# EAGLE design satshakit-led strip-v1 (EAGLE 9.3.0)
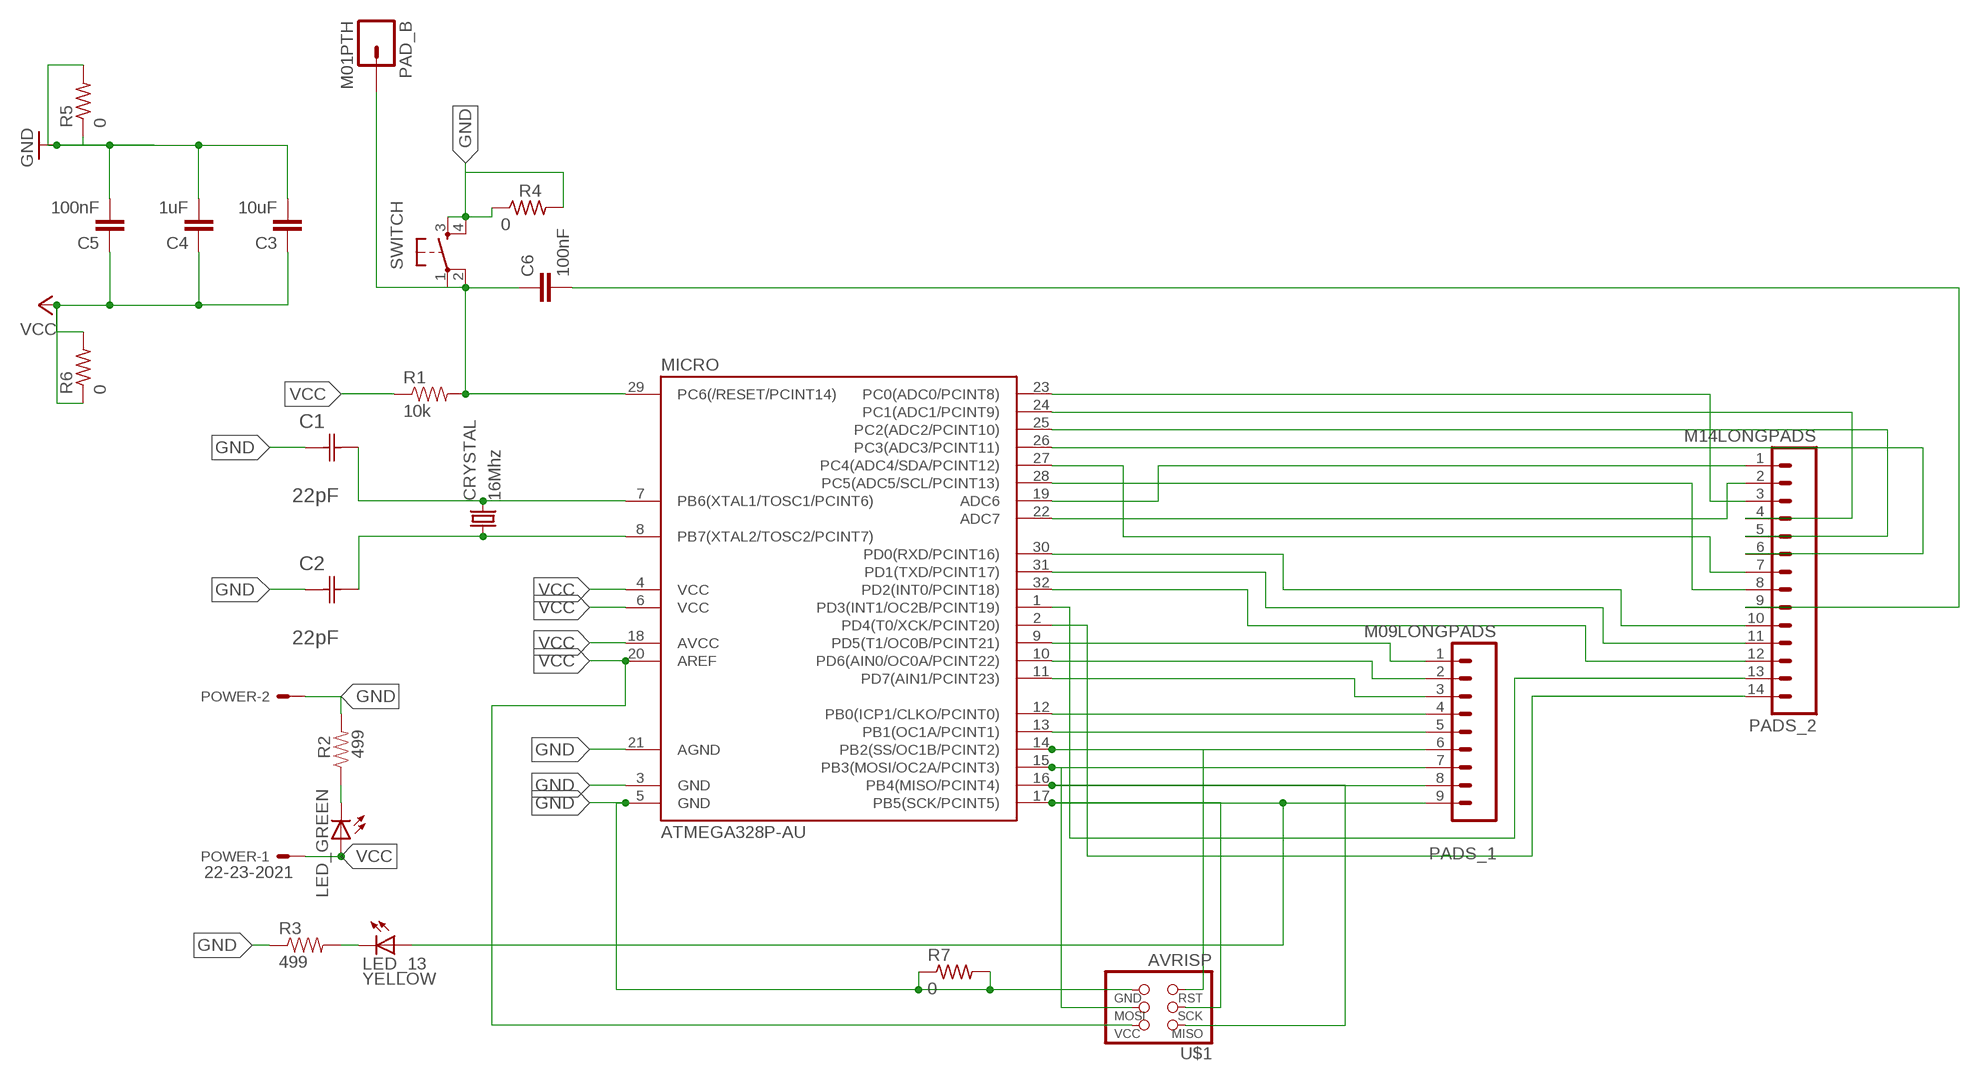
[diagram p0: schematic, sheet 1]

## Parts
C1  22pF  0612ZC225MAT2A  [CAPC3216X178N]
C2  22pF  0612ZC225MAT2A  [CAPC3216X178N]
C3  10uF  CAP1206  [1206]
C4  1uF  CAP1206  [1206]
C5  100nF  CAP1206  [1206]
C6  100nF  CAP1206  [1206]
CRYSTAL  16Mhz  CSM-7X-DU  [CSM-7X-DU]
LED_13  YELLOW  LED1206  [1206]
LED_GREEN  LED1206  [1206]
MICRO  ATMEGA328P-AU  ATMEGA48/88/168-AU  [TQFP32-08]
PAD_B  M01PTH  [1X01]
PADS_1  M09LONGPADS  [1X09_LONGPADS]
PADS_2  M14LONGPADS  [1X14-LONGPADS]
POWER  22-23-2021  [22-23-2021]
R1  10k  RESISTOR1206  [1206]
R2  499  RESISTOR1206  [1206]
R3  499  RESISTOR1206  [1206]
R4  0  RES-US1206  [R1206]
R5  0  RES-US1206FAB  [R1206FAB]
R6  0  RES-US1206FAB  [R1206FAB]
R7  0  RES-US1206FAB  [R1206FAB]
SWITCH  6MM_SWITCH6MM_SWITCH  [6MM_SWITCH]
U$1  AVRISP  [2X03]

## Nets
GND: C1.1(C1) C2.1(C1) C3.2 C4.2 C5.2 MICRO.3(GND) MICRO.5(GND) MICRO.21(AGND) POWER.2 R2.2 R3.1 R4.1 R4.2 R5.1 R5.2 R7.1 R7.2 SWITCH.3(S) SWITCH.4(S1) U$1.6(GND)
N$1: MICRO.9(PD5(T1/OC0B/PCINT21)) PADS_1.1
N$2: C1.2(C2) CRYSTAL.2 MICRO.7(PB6(XTAL1/TOSC1/PCINT6))
N$3: C6.2 PADS_2.9
N$4: MICRO.10(PD6(AIN0/OC0A/PCINT22)) PADS_1.2
N$5: MICRO.11(PD7(AIN1/PCINT23)) PADS_1.3
N$6: MICRO.12(PB0(ICP1/CLKO/PCINT0)) PADS_1.4
N$7: MICRO.13(PB1(OC1A/PCINT1)) PADS_1.5
N$8: MICRO.14(PB2(SS/OC1B/PCINT2)) PADS_1.6 U$1.5(RST)
N$9: C2.2(C2) CRYSTAL.1 MICRO.8(PB7(XTAL2/TOSC2/PCINT7))
N$10: MICRO.15(PB3(MOSI/OC2A/PCINT3)) PADS_1.7 U$1.4(MOSI)
N$11: MICRO.16(PB4(MISO/PCINT4)) PADS_1.8 U$1.1(MISO)
N$12: LED_13.1(A) MICRO.17(PB5(SCK/PCINT5)) PADS_1.9 U$1.3(SCK)
N$13: MICRO.19(ADC6) PADS_2.1
N$14: MICRO.22(ADC7) PADS_2.2
N$15: MICRO.23(PC0(ADC0/PCINT8)) PADS_2.3
N$16: MICRO.24(PC1(ADC1/PCINT9)) PADS_2.4
N$17: MICRO.25(PC2(ADC2/PCINT10)) PADS_2.5
N$18: MICRO.26(PC3(ADC3/PCINT11)) PADS_2.6
N$19: MICRO.27(PC4(ADC4/SDA/PCINT12)) PADS_2.7
N$20: MICRO.30(PD0(RXD/PCINT16)) PADS_2.10
N$21: MICRO.31(PD1(TXD/PCINT17)) PADS_2.11
N$22: MICRO.32(PD2(INT0/PCINT18)) PADS_2.12
N$23: MICRO.1(PD3(INT1/OC2B/PCINT19)) PADS_2.13
N$24: MICRO.2(PD4(T0/XCK/PCINT20)) PADS_2.14
N$25: MICRO.28(PC5(ADC5/SCL/PCINT13)) PADS_2.8
N$26: LED_GREEN.2(C) R2.1
N$27: LED_13.2(C) R3.2
N$28: C6.1 MICRO.29(PC6(/RESET/PCINT14)) PAD_B.1 R1.2 SWITCH.1(P) SWITCH.2(P1)
VCC: C3.1 C4.1 C5.1 LED_GREEN.1(A) MICRO.4(VCC) MICRO.6(VCC) MICRO.18(AVCC) MICRO.20(AREF) POWER.1 R1.1 R6.1 R6.2 U$1.2(VCC)

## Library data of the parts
C1 C2 = AVX_By_element14_Batch_1:0612ZC225MAT2A: Capacitor 1206; MPN: 0612ZC225MAT2A; OC_FARNELL: -; OC_NEWARK: 12N3209; SUPPLIER: AVX; TOLERANCE: ±20%; VALUE: 2.2µF; VOLTAGERATING: 10V
C3-C6 = 01_SparkFun:CAP: Capacitor
CRYSTAL = 01_FAB_Hello:CSM-7X-DU: SMD CRYSTAL; OC_FARNELL: unknown; OC_NEWARK: unknown
LED_13 LED_GREEN = 01_FAB_Hello:LED
MICRO = atmega8:ATMEGA48/88/168
PAD_B = 01_SparkFun:M01: Header 1
PADS_1 = 01_SparkFun:M09: Header 9 Standard 9-pin 0.1" header. Use with straight break away headers (SKU : PRT-00116), right angle break away headers (PRT-00553), swiss pins (PRT-00743), machine pins (PRT-00117), and female headers (PRT-00115).
PADS_2 = 01_SparkFun:M14: Header 14 Standard 14-pin 0.1" header. Use with straight break away headers (SKU : PRT-00116), right angle break away headers (PRT-00553), swiss pins (PRT-00743), machine pins (PRT-00117), and female headers (PRT-00115).
POWER = con-molex:22-23-2021: .100" (2.54mm) Center Header - 2 Pin; MF: MOLEX; MPN: 22-23-2021; OC_FARNELL: 1462926; OC_NEWARK: 25C3832
R1-R3 = 01_SparkFun:RESISTOR: Resistor
R4-R7 = fab:RES-US: Resistor (US Symbol)
SWITCH = 01_FAB_Hello:6MM_SWITCH: OMRON SWITCH
U$1 = fab:AVRISP

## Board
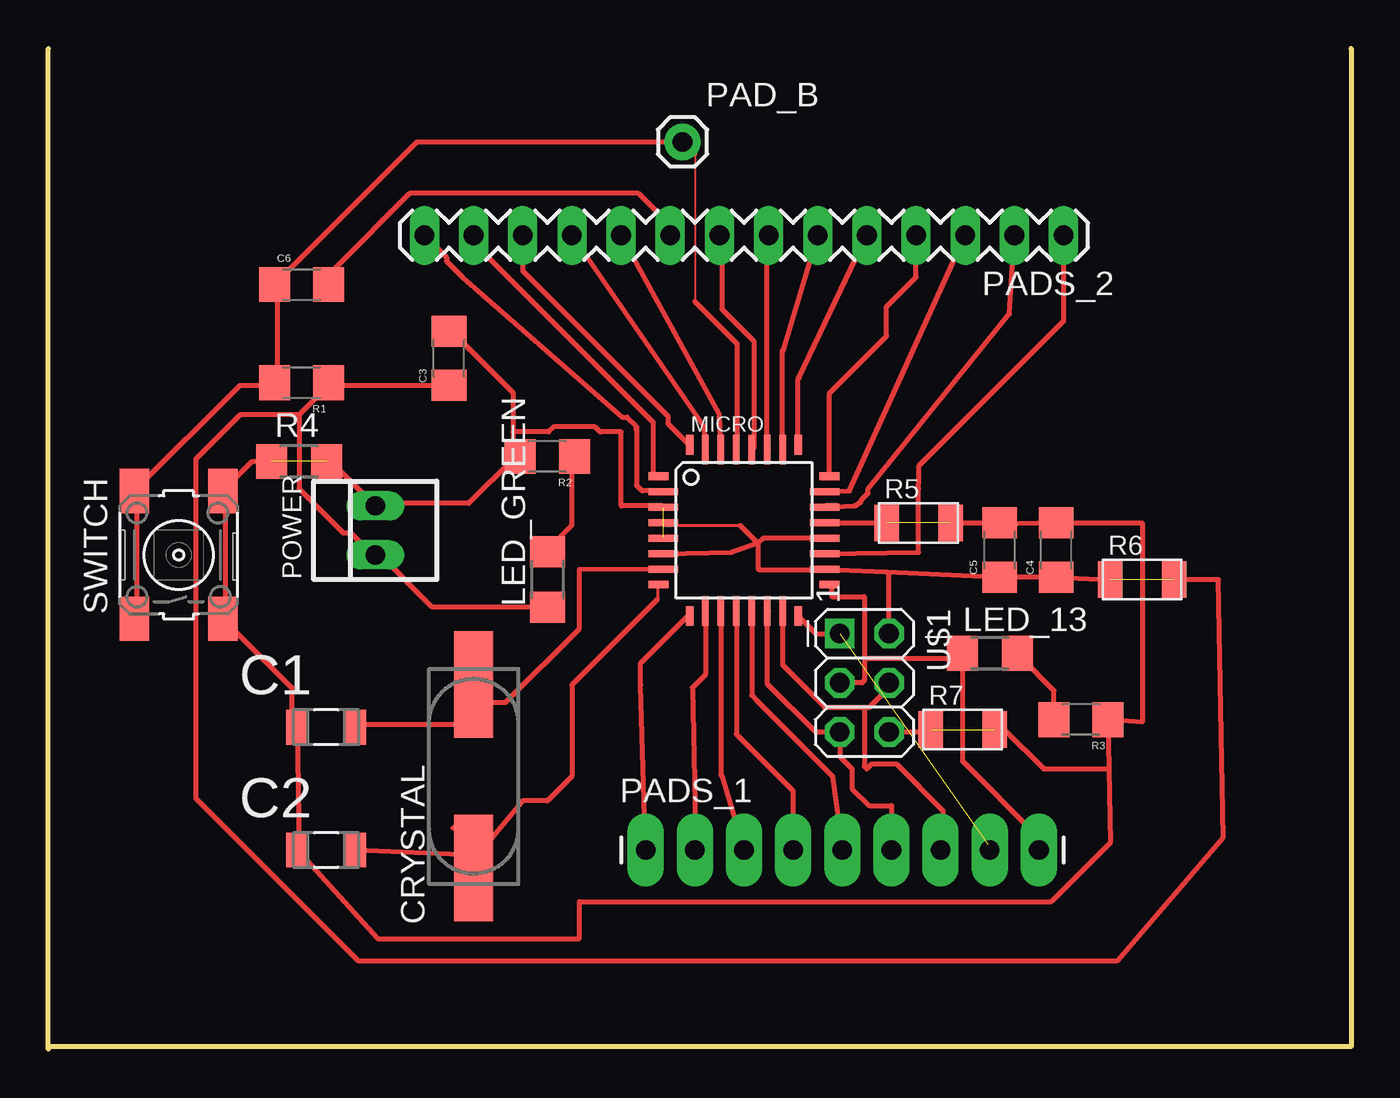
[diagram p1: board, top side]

Size 67.31 x 51.69 mm. Coordinates in mm from the lower left corner, seen from the top.
Outline: 0,0 0,51.69
Outline: 67.31,51.69 67.31,0.13 0.13,0.13
Copper layers (1*16): Top 0.035mm / dielectric 1.5mm / Bottom 0.035mm
Design rules "default *": minimum track width 10mil, minimum drill 0.35mm, track to track 16mil, track to pad 20mil, pad to pad 20mil, via to via 20mil, smd to smd 20mil, copper to edge 40mil, drill to drill 6mil, minimum pad ring 10mil, minimum via ring 8mil, stop-mask expansion 4mil, vias tented up to drill 0mil, thermal gap 10mil

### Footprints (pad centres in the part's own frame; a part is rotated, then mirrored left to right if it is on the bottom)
CAPC3216X178N = smd 1.118 x 1.803: 1 -1.499,0; 2 1.499,0
1206 = smd 1.6 x 1.8: 1 -1.4,0; 2 1.4,0
CSM-7X-DU = smd 5.5 x 2: 1 -4.75,0; 2 4.75,0
1206' = smd 1.6 x 1.803: 1 -1.422,0; 2 1.422,0
TQFP32-08 = smd 1.016 x 0.406: 1 -4.42,2.8; 8 -4.42,-2.8; 17 4.42,-2.8; 24 4.42,2.8 | smd 1.524 x 0.356: 2 -4.166,2; 3 -4.166,1.2; 4 -4.166,0.4; 5 -4.166,-0.4; 6 -4.166,-1.2; 7 -4.166,-2; 18 4.166,-2; 19 4.166,-1.2; 20 4.166,-0.4; 21 4.166,0.4; 22 4.166,1.2; 23 4.166,2 | smd 0.406 x 1.016: 9 -2.8,-4.42; 16 2.8,-4.42; 25 2.8,4.42; 32 -2.8,4.42 | smd 0.356 x 1.524: 10 -2,-4.166; 11 -1.2,-4.166; 12 -0.4,-4.166; 13 0.4,-4.166; 14 1.2,-4.166; 15 2,-4.166; 26 2,4.166; 27 1.2,4.166; 28 0.4,4.166; 29 -0.4,4.166; 30 -1.2,4.166; 31 -2,4.166
1X01 = drill 1.016 pad 1.88: 1 0,0
1X09_LONGPADS = drill 1.016 pad 1.88 long: 1 0,0; 2 2.54,0; 3 5.08,0; 4 7.62,0; 5 10.16,0; 6 12.7,0; 7 15.24,0; 8 17.78,0; 9 20.32,0
1X14-LONGPADS = drill 1.016 long: 1 0,0; 2 2.54,0; 3 5.08,0; 4 7.62,0; 5 10.16,0; 6 12.7,0; 7 15.24,0; 8 17.78,0; 9 20.32,0; 10 22.86,0; 11 25.4,0; 12 27.94,0; 13 30.48,0; 14 33.02,0
22-23-2021 = drill 1 long: 1 -1.27,0; 2 1.27,0
R1206 = smd 1.6 x 1.803: 1 -1.422,0; 2 1.422,0
R1206FAB = smd 1.27 x 1.905: 1 -1.651,0; 2 1.651,0
6MM_SWITCH = smd 2.286 x 1.524: 1 -3.302,2.286; 2 3.302,2.286; 3 -3.302,-2.286; 4 3.302,-2.286
2X03 = drill 1.016 square: 1 -2.54,-1.27 | drill 1.016 octagon: 2 -2.54,1.27; 3 0,-1.27; 4 0,1.27; 5 2.54,-1.27; 6 2.54,1.27

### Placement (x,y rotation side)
C1  14.35,16.64 0 top
C2  14.35,10.29 0 top
C3  20.7,35.69 90 top
C4  52.07,25.78 90 top
C5  49.15,25.78 90 top
C6  13.08,39.5 0 top
CRYSTAL  21.97,14.1 90 top
LED_13  YELLOW  [1206']  48.64,20.45 0 top
LED_GREEN  [1206']  25.78,24.26 90 top
MICRO  35.94,26.8 0 top
PAD_B  32.77,46.86 0 top
PADS_1  30.86,10.29 0 top
PADS_2  52.45,42.04 180 top
POWER  16.89,26.8 90 top
R1  13.08,34.42 180 top
R2  25.78,30.61 180 top
R3  53.34,17.02 180 top
R4  12.95,30.35 0 top
R5  44.96,27.18 0 top
R6  56.52,24.26 0 top
R7  47.24,16.51 0 top
SWITCH  6.73,25.53 90 top
U$1  42.16,18.92 270 top

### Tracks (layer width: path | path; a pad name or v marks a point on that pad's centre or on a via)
GND  (4 unrouted)
  Top 0.152: 31.17,26.44 31.77,26.44 MICRO.5 31.77,26.29 | 40.01,27.2 MICRO.21 40.16,27.2 41.07,27.2
  Top 0.254: 52.45,27.18 52.33,27.18 | 52.33,27.18 C4.2 49.15,27.11 C5.2 R5.2 | 12.95,16.38 C1.1 | C1.1 12.57,16.76 12.57,18.67 SWITCH.3 9.14,22.48 9.14,28.57 SWITCH.4 10.54,30.35 R4.1 | 24,31.88 24,33.91 20.95,36.96 C3.2 | 24,31.88 24,30.86 R2.2 24,30.48 21.72,28.19 17.14,28.19 POWER.2 15.01,29.95 R4.2 | 31.77,27.96 MICRO.3 31.7,28.07 29.59,28.07 29.59,31.88 28.51,31.88 28.24,32.14 26.12,32.14 25.85,31.88 24,31.88 | MICRO.21 R5.1 | 52.33,27.18 54.86,27.18 56.52,27.18 56.52,16.89 R3.1 54.79,14.48 | 54.79,14.48 54.86,10.67 51.82,7.62 27.43,7.62 27.43,5.71 17.02,5.71 C2.1 12.95,10.29 C1.1 | U$1.6 45.47,16.38 R7.1 | R7.2 49.4,16.51 51.44,14.48 54.79,14.48
N$1
  Top 0.152: PADS_1.1 30.86,10.44 | 32.99,22.33 MICRO.9
  Top 0.254: PADS_1.1 30.61,18.8 30.61,19.94 32.99,22.33
N$2
  Top 0.152: 31.77,24.77 MICRO.7 | 22.07,18.92 CRYSTAL.2 21.92,18.77
  Top 0.254: C1.2 16,16.76 20.95,16.76 21.7,17.51 CRYSTAL.2 22.33,17.91 23.62,17.91 27.43,21.72 27.43,24.77 MICRO.7
N$3
  Top 0.152: 32.08,42.14 PADS_2.9
  Top 0.254: C6.2 14.86,39.62 14.86,40.39 18.67,44.2 30.48,44.2 32.38,42.29 PADS_2.9
N$4
  Top 0.152: 33.91,10.74 33.45,10.29 PADS_1.2 | 33.91,22.63 MICRO.10
  Top 0.254: 33.45,10.29 33.27,18.67 33.94,19.34 MICRO.10
N$5
  Top 0.152: 34.82,22.63 MICRO.11 | 35.89,10.29 PADS_1.3
  Top 0.254: PADS_1.3 34.8,14.1 34.74,14.15 MICRO.11
N$6
  Top 0.152: PADS_1.4 38.48,10.44 | 35.59,22.63 MICRO.12
  Top 0.254: PADS_1.4 38.48,13.34 35.54,16.27 MICRO.12
N$7
  Top 0.152: 40.92,10.59 40.92,10.29 PADS_1.5 | MICRO.13
  Top 0.254: PADS_1.5 40.51,14.1 36.77,17.84 36.58,18.03 36.34,18.27 MICRO.13
N$8
  Top 0.152: 37.26,22.63 MICRO.14 | 43.66,10.29 PADS_1.6
  Top 0.254: MICRO.14 37.14,18.87 39.62,16.38 U$1.5 40.89,15.11 41.53,14.48 41.53,13.46 42.42,12.57 43.56,12.57 43.56,10.39 43.66,10.29
N$9
  Top 0.152: 31.47,23.24 31.47,23.85 MICRO.8
  Top 0.254: 20.9,11.43 21.84,11.43 CRYSTAL.1 | 31.47,23.24 27.05,18.82 27.05,14.1 25.78,12.83 24.51,12.83 21.97,9.78 | 21.97,10.29 21.97,10.03 | 21.97,10.03 21.97,9.78 | 21.97,9.78 CRYSTAL.1 | CRYSTAL.1 21.5,9.82 | CRYSTAL.1 21.64,9.35 | C2.2 21.97,10.03
N$10
  Top 0.152: PADS_1.7 46.1,10.44 | 38.02,22.63 MICRO.15
  Top 0.254: MICRO.15 37.94,19.84 40.13,17.65 42.16,17.65 | U$1.4 43.43,18.67 42.42,17.65 42.16,17.65 | 42.16,17.65 42.16,14.61 42.29,14.48 42.55,14.73 43.81,14.73 46.23,12.32 46.23,10.41 PADS_1.7
N$11  (1 unrouted)
  Top 0.152: 48.54,10.59 48.54,10.29 PADS_1.8 | 38.79,22.33 MICRO.16
  Top 0.254: MICRO.16 39.66,21.46 U$1.1
N$12  (1 unrouted)
  Top 0.152: 51.13,10.29 PADS_1.9
  Top 0.254: 47.24,20.19 47.24,14.86 51.05,11.05 51.05,10.29 PADS_1.9 | 47.24,20.19 47.22,20.43 LED_13.1 | 40.36,23.98 40.46,23.88 40.46,23.39 40.49,23.37 42.16,23.37 42.16,20.19 | 42.16,20.19 42.16,19.05 42.04,18.92 U$1.3 | 42.16,20.19 47.24,20.19
N$13
  Top 0.152: 40.77,25.68 40.16,25.68 MICRO.19
  Top 0.254: MICRO.19 44.96,25.65 44.96,28.96 44.96,29.21 44.96,30.1 52.45,37.59 PADS_2.1
N$14
  Top 0.152: 40.77,28.12 40.16,28.12 MICRO.22 | 49.91,41.07 PADS_2.2
  Top 0.254: MICRO.22 41.66,28.07 41.74,28.07 41.83,28.18 41.97,28.23 42.04,28.4 42.35,28.7 42.35,28.93 49.66,37.97 PADS_2.2
N$15
  Top 0.152: 40.77,28.88 40.16,28.88 MICRO.23
  Top 0.254: MICRO.23 41.4,28.83 PADS_2.3
N$16
  Top 0.152: 40.46,29.64 MICRO.24
  Top 0.254: MICRO.24 40.36,33.88 43.31,36.83 43.31,38.35 44.83,39.88 PADS_2.4
N$17
  Top 0.152: 38.79,31.32 MICRO.25
  Top 0.254: PADS_2.5 38.79,34.67 38.74,34.63 MICRO.25
N$18
  Top 0.152: 38.02,31.01 MICRO.26
  Top 0.254: 37.97,36.07 38.01,36.19 | 38.01,36.19 PADS_2.6 | MICRO.26 37.94,36.12 38.01,36.19
N$19
  Top 0.152: 37.26,31.01 MICRO.27
  Top 0.254: MICRO.27 37.14,41.97 PADS_2.7
N$20
  Top 0.152: 34.67,31.01 MICRO.30
  Top 0.254: MICRO.30 34.67,32.77 PADS_2.10
N$21
  Top 0.152: 33.91,31.01 MICRO.31
  Top 0.254: MICRO.31 33.91,32.13 PADS_2.11
N$22
  Top 0.152: 32.99,31.32 MICRO.32
  Top 0.254: PADS_2.12 24.51,40.19 32,32.7 32,32.31 32.99,31.32
N$23
  Top 0.152: 31.47,29.64 MICRO.1 | 21.87,41.99 PADS_2.13
  Top 0.254: MICRO.1 31.24,29.72 31.24,32.38 21.72,41.91 PADS_2.13
N$24
  Top 0.152: 31.77,28.88 MICRO.2 | 19.43,41.99 PADS_2.14
  Top 0.254: PADS_2.14 20.57,40.89 20.57,40.7 21.39,39.88 29.65,32.64 29.91,32.64 30.35,32.19 30.35,32.03 30.38,32 | 30.38,32.17 30.38,32 | 30.38,32 30.38,29.13 30.68,28.83 31.74,28.83 MICRO.2
N$25
  Top 0.152: 36.35,31.01 MICRO.28
  Top 0.254: PADS_2.8 34.8,41.91 34.8,38.23 36.45,36.58 36.45,31.07 MICRO.28
N$26
  Top 0.254: R2.1 27.05,30.48 27.05,27.05 25.91,25.91 LED_GREEN.2
N$27
  Top 0.254: R3.2 51.95,18.51 50.29,20.19 LED_13.2
N$28
  Top 0.102: 33.4,46.23 33.4,38.61
  Top 0.152: 35.59,31.01 MICRO.29
  Top 0.254: SWITCH.1 4.57,22.48 4.57,28.57 SWITCH.2 9.91,34.29 11.43,34.29 R1.2 11.81,34.67 11.81,39.24 C6.1 11.81,39.62 19.05,46.86 PAD_B.1 33.4,46.23 | 35.59,31.01 35.59,36.42 33.4,38.61
VCC  (1 unrouted)
  Top 0.152: 40.01,26.29 MICRO.20 | 35.74,27.05 31.77,27.05 MICRO.4 | 40.16,24.77 MICRO.18 | 31.77,25.53 MICRO.6
  Top 0.254: LED_GREEN.1 25.53,22.86 19.81,22.86 17.14,25.53 POWER.1 16.76,25.53 15.62,26.67 15.24,26.67 12.95,28.96 12.95,32.77 | 49.4,24.51 C5.1 | 51.94,24.51 C4.1 | C3.1 20.57,34.29 14.86,34.29 R1.1 14.48,34.29 12.95,32.77 | 12.95,32.77 9.91,32.77 7.62,30.48 7.62,12.95 16,4.57 55.24,4.57 60.71,10.92 60.45,24.26 R6.2 | 49.02,24.51 C5.1 | C4.1 49.4,24.38 | 49.4,24.38 C5.1 | MICRO.6 35.31,25.65 36.66,26.12 | C4.1 R6.1 | 43.31,24.65 MICRO.18 40.08,24.77 36.7,24.77 36.66,24.8 36.66,26.12 | 43.31,24.65 49.4,24.38 | 35.74,27.05 36.66,26.12 | MICRO.20 36.94,26.4 36.66,26.12 | U$1.2 43.43,24.53 43.31,24.65
~_REAL_OUTLINEMILL_~  (via drill 0.3 pad 0.5)
  other vias: -5.02,-5.02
